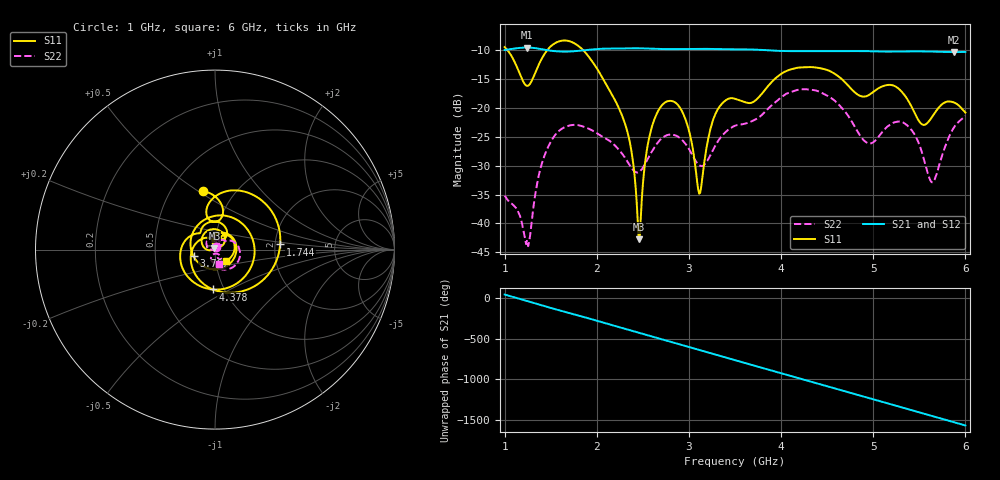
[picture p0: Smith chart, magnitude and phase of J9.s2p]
!Agilent Technologies,E8364B,MY43040528,A.07.50.67
!Agilent E8364B: A.07.50.67
!Date: Sunday, March 01, 2026 18:33:46
!Correction: S11(Full 2 Port(1,2))
!S21(Full 2 Port(1,2))
!S12(Full 2 Port(1,2))
!S22(Full 2 Port(1,2))
!S2P File: Measurements: S11, S21, S12, S22:
# Hz S  dB  R 50
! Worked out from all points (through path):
!   451 points, 1 GHz to 6 GHz, reference 50 ohm
!   highest |S21| = -9.60 dB at 1.244 GHz (marker M1); lowest = -10.4 dB at 5.878 GHz (marker M2)
!   group delay of S21, straight-line fit = 897 ps
!   lowest |S11| = -42.7 dB at 2.456 GHz (marker M3), VSWR 1.01, Z = 49.7 + j0.644 ohm
!   |S11| at or under -10 dB: 1.028 GHz to 1.466 GHz (437.2 MHz wide, 35.1 % of centre); 1.849 GHz to end of sweep
!   |S22| runs from -43.9 to -16.8 dB; largest |S21 - S12| = 0.0013
!   S11 on the Smith chart (normalised r, x): 1 GHz: 0.71, +0.52; 1.744 GHz: 2.13, +0.14; 3.767 GHz: 0.78, -0.06; 4.378 GHz: 0.88, -0.41; 6 GHz: 1.12, -0.15
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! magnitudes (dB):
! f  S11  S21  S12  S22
! 1 GHz  -9.5  -10.0  -10.1  -35.2
! 1.244 GHz  -16.2  -9.6  -9.6  -42.9
! 1.444 GHz  -10.4  -10.0  -10.0  -27.8
! 1.744 GHz  -8.8  -10.3  -10.3  -23.0
! 1.844 GHz  -9.9  -10.1  -10.1  -23.2
! 2.311 GHz  -23.0  -9.8  -9.8  -28.8
! 2.456 GHz  -42.7  -9.7  -9.8  -31.1
! 2.556 GHz  -26.2  -9.8  -9.8  -28.8
! 2.667 GHz  -20.5  -9.8  -9.9  -25.9
! 2.922 GHz  -20.5  -9.9  -9.9  -25.5
! 3.111 GHz  -34.9  -9.8  -9.8  -29.9
! 3.278 GHz  -21.4  -9.9  -9.9  -26.8
! 3.5 GHz  -18.5  -9.9  -9.9  -23.1
! 3.767 GHz  -18.0  -10.0  -10.0  -21.6
! 4.344 GHz  -13.0  -10.2  -10.2  -16.9
! 4.378 GHz  -13.1  -10.2  -10.2  -17.0
! 4.933 GHz  -18.0  -10.2  -10.2  -26.1
! 5.167 GHz  -16.1  -10.3  -10.3  -23.1
! 5.411 GHz  -19.7  -10.3  -10.3  -23.8
! 5.644 GHz  -21.4  -10.3  -10.3  -32.9
! 5.878 GHz  -19.1  -10.4  -10.4  -23.4
! 6 GHz  -20.8  -10.4  -10.4  -21.4
